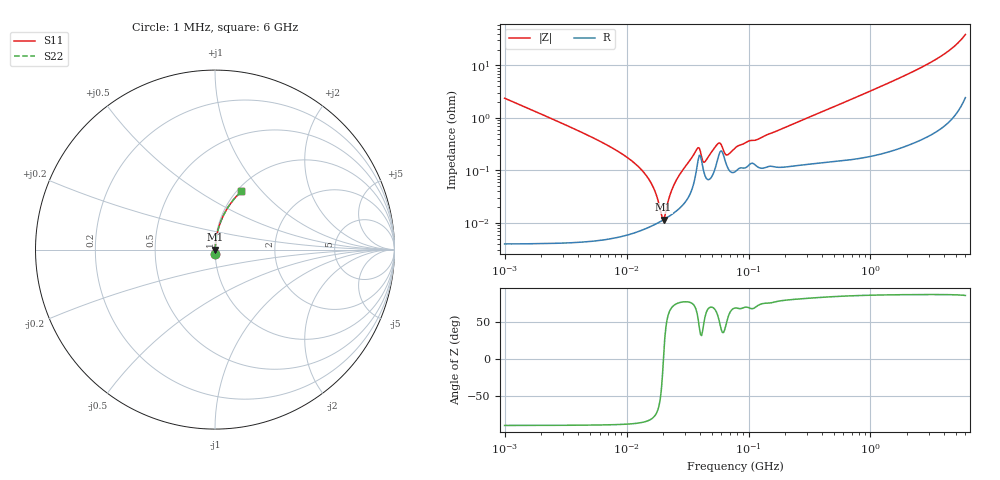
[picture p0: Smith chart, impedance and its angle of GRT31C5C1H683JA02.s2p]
!Murata Part Number: GRT31C5C1H683JA02
!These Parameters are Measured in Series Mode Connection
!Data Generated on Jun 19, 2026
!  o--ll--o
!Port1  Port2
!  o------o
!Operation Temp=25[degC], DC Bias Voltage=0[V]
!Freq. Start=1000[kHz] Stop=6[GHz] 401[Steps]
# Hz S RI R 50
!Freq.(Hz) S11(Real) S11(Imag) S21(Real) S21(Imag) S12(Real) S12(Imag) S22(Real) S22(Imag)
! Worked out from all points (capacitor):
!   401 points, 1 MHz to 6 GHz, reference 50 ohm
!   read as one part in series: C = 66.6 nF near 1.044 MHz
!   lowest |Z| = 11.5 mohm at 20.11 MHz (marker M1)
!   series resonance near 20.05 MHz, so ESL is about 950 pH
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1000000  0.000608 -0.0238  0.9994 0.0238  0.9994 0.0238  0.000608 -0.0238
4293785  7.14e-05 -0.00532  0.9999 0.00532  0.9999 0.00532  7.14e-05 -0.00532
8245209  5.83e-05 -0.00242  0.9999 0.00242  0.9999 0.00242  5.83e-05 -0.00242
1.219603e7  6.89e-05 -0.00125  0.9999 0.00125  0.9999 0.00125  6.89e-05 -0.00125
1.583299e7  8.65e-05 -0.00058  0.9999 0.00058  0.9999 0.00058  8.65e-05 -0.00058
1.727208e7  9.51e-05 -0.000366  0.9999 0.000366  0.9999 0.000366  9.51e-05 -0.000366
1.843659e7  0.000103 -0.000206  0.9999 0.000206  0.9999 0.000206  0.000103 -0.000206
1.925624e7  0.000109 -9.97e-05  0.9999 9.97e-05  0.9999 9.97e-05  0.000109 -9.97e-05
2.011232e7  0.000115 7.4e-06  0.9999 -7.4e-06  0.9999 -7.4e-06  0.000115 7.4e-06
2.291577e7  0.00014 0.000336  0.9999 -0.000336  0.9999 -0.000336  0.00014 0.000336
2.499862e7  0.000162 0.000568  0.9998 -0.000568  0.9998 -0.000568  0.000162 0.000568
3.779011e7  0.00117 0.00227  0.9988 -0.00227  0.9988 -0.00227  0.00117 0.00227
3.947016e7  0.00194 0.00182  0.9981 -0.00182  0.9981 -0.00182  0.00194 0.00182
4.400437e7  0.000792 0.00124  0.9992 -0.00124  0.9992 -0.00124  0.000792 0.00124
5.589783e7  0.00164 0.00276  0.9984 -0.00276  0.9984 -0.00276  0.00164 0.00276
5.838291e7  0.00226 0.00242  0.9977 -0.00242  0.9977 -0.00242  0.00226 0.00242
6.652088e7  0.00122 0.00154  0.9988 -0.00154  0.9988 -0.00154  0.00122 0.00154
7.745967e7  0.000949 0.0025  0.9991 -0.0025  0.9991 -0.0025  0.000949 0.0025
3.325952e8  0.00145 0.0109  0.9985 -0.0109  0.9985 -0.0109  0.00145 0.0109
1.428092e9  0.00447 0.0468  0.9955 -0.0468  0.9955 -0.0468  0.00447 0.0468
3.5601e9  0.0238 0.1332  0.9762 -0.1332  0.9762 -0.1332  0.0238 0.1332
6e9  0.1469 0.324  0.8531 -0.324  0.8531 -0.324  0.1469 0.324
